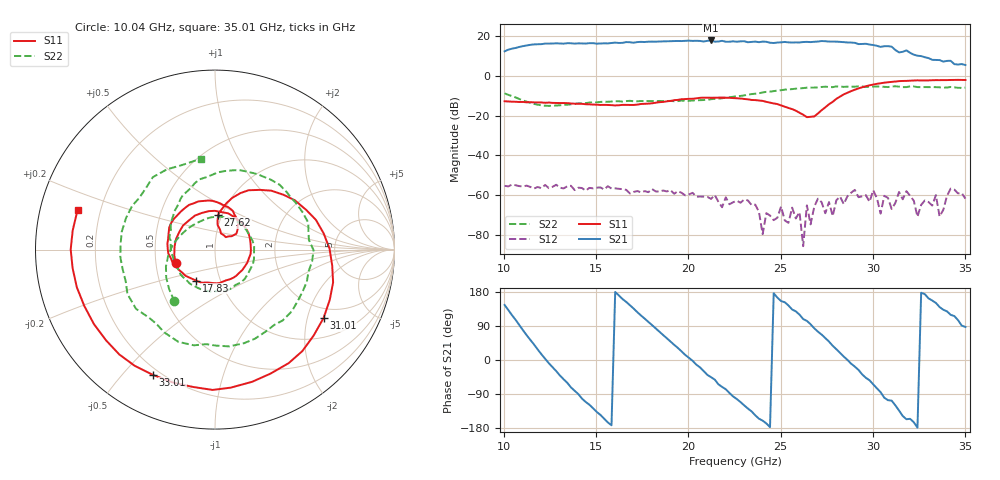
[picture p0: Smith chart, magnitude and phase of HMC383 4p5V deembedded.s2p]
!Hittite Microwave Corporation
!20 Alpha Road
!Chelmsford, MA 01824
!Tel: 978-250-3343
!Fax: 978-250-3373
!Device: HMC383, 12-30 GHz, Driver Amplifier Die
!Misc: Vcc = 4.5V, data includes two K connectors, Room
# MHZ S MA R 50
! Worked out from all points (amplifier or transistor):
!   126 points, 10.04 GHz to 35.01 GHz, reference 50 ohm
!   highest |S21| = 18.0 dB at 21.22 GHz (marker M1)
!   |S21| within 3 dB of that: 10.97 GHz to 30.32 GHz (19.35 GHz wide, 93.7 % of centre)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
!   unconditionally stable (mu >= 1): start of sweep to end of sweep
!   at 14.23 GHz: K = 45.85, MAG = 16.9 dB, |S12| = -56.5 dB
!   at 22.62 GHz: K = 79.18, MAG = 18.1 dB, |S12| = -62.9 dB
!   at 35.01 GHz: K = 87.37, MAG = 11.3 dB, |S12| = -61.8 dB
!   S11 on the Smith chart (normalised r, x): 10.04 GHz: 0.63, -0.10; 17.83 GHz: 0.77, -0.28; 27.62 GHz: 0.96, +0.39; 31.01 GHz: 1.62, -2.53; 33.01 GHz: 0.17, -0.61; 35.01 GHz: 0.12, +0.14
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10037.5  0.232 -161.1  4.215 145.3  0.001702 -16.8  0.366 -128.1
11036.25  0.223 143.0  5.697 78.4  0.00165 -27.1  0.243 177.3
12234.75  0.212 79.3  6.606 3.2  0.001796 -43.1  0.179 123.6
13433.25  0.208 25.7  6.766 -60.1  0.001662 -65.2  0.19 68.7
14232.25  0.2 -6.6  6.676 -102.0  0.001503 -77.1  0.206 31.4
16030  0.182 -69.8  6.988 179.6  0.001472 -89.4  0.233 -45.0
16829  0.187 -92.9  7.151 144.5  0.001094 -113.3  0.238 -74.6
17827.75  0.202 -121.2  7.38 100.5  0.001182 -114.2  0.235 -107.8
18427  0.22 -138.6  7.448 74.6  0.001221 -116.2  0.236 -126.0
20025  0.267 173.2  7.836 5.8  0.001035 -140.0  0.237 -168.9
21223.5  0.284 137.3  7.925 -45.3  0.0007989 -142.6  0.261 166.2
22621.75  0.276 97.7  7.351 -103.1  0.0007173 -148.1  0.311 136.5
24219.75  0.224 61.4  7.33 -167.4  0.0003488 154.3  0.401 102.4
25218.5  0.169 41.8  7.265 152.4  0.0002281 65.1  0.455 76.4
26816.5  0.096 69.8  7.342 83.7  0.0005056 -64.4  0.513 34.5
27615.5  0.195 84.9  7.428 48.5  0.0006627 -104.4  0.53 10.9
29013.75  0.454 46.3  6.913 -17.4  0.001348 -104.5  0.542 -30.8
30012.5  0.612 8.5  6.071 -64.4  0.001319 -130.3  0.544 -65.8
31011.25  0.715 -32.2  5.515 -107.2  0.0004435 -106.6  0.546 -102.4
31810.25  0.757 -65.8  4.453 -156.3  0.001252 -177.5  0.528 -133.9
33008.75  0.779 -116.4  2.847 162.7  0.0006655 75.6  0.527 176.9
35006.25  0.797 163.9  1.904 87.1  0.0008088 72.4  0.513 99.0
